|   stm32f0_448_lqfp100 IBIS Model
[IBIS ver]   4.2
[File name]  stm32f0_448_lqfp100.ibs
[File Rev]   1.0
[Date]   15-5-2013
[Source] Data Created at STMicroelectronics
[Notes]   File originated from ELDO simulations.
[Disclaimer]  This information is for modeling purpose only and is
   not guaranted. The information is subject to change without
   notice.
[Copyright] Copyright 2015 STMicroelectronics Inc.
[Component] stm32f0_448_lqfp100
[Manufacturer] STMicroelectronics
[Package]
| variable   typ   min   max
R_pkg   0.0   NA   NA
L_pkg   0.0H   NA   NA
C_pkg   0.0F   NA   NA
[Pin] signal_name  model_name   R_pin   L_pin   C_pin
1   PE2   io8p_sudq_ft   0.132430474   7.03E-09   1.35E-13
2   PE3   io8p_sudq_ft   0.133347678   6.77E-09   1.95E-14
3   PE4   io8p_sudq_ft   0.12897311   6.49E-09   1.04E-14
4   PE5   io8p_sudq_ft   0.125344562   6.21E-09   5.24E-15
5   PE6   io8p_sudq_ft   0.120515446   5.99E-09   7.82E-15
6   VBAT   POWER   0.12047071   5.95E-09   6.53E-15
7   PC13   io8p_sudq_tc   0.117880646   5.78E-09   6.23E-15
8   PC14   io8p_sudq_tc   0.117278614   5.65E-09   3.11E-15
9   PC15   io8p_sudq_tc   0.11554812   5.55E-09   1.39E-15
10   PF9   io8p_sudq_ft   0.114995632   5.43E-09   2.92E-15
11   PF10   io8p_sudq_ft   0.112975638   5.30E-09   3.56E-15
12   PF0   io8p_sudq_ft   0.111323436   5.23E-09   4.78E-15
13   PF1   io8p_sudq_ft   0.109216856   5.14E-09   8.66E-15
14   NRST   ioreset_tc_v33   0.11066442   5.18E-09   9.03E-15
15   PC0   io8p_sudq_ft   0.110607546   5.19E-09   7.98E-15
16   PC1   io8p_sudq_ft   0.111326184   5.25E-09   1.03E-14
17   PC2   io8p_sudq_ft   0.11442005   5.35E-09   7.00E-15
18   PC3   io8p_sudq_ft   0.114363236   5.45E-09   8.65E-15
19   PF2   io8p_sudq_ft   0.117563732   5.62E-09   7.83E-15
20   VSSA   GND   0.119904688   5.80E-09   2.29E-16
21   VDDA   POWER   0.122311852   5.96E-09   1.05E-15
22   PF3   io8p_sudq_ft   0.125384354   6.19E-09   8.12E-16
23   PA0   io8p_sudq_ft   0.129702038   6.49E-09   3.82E-15
24   PA1   io8p_sudq_ft   0.13229018   6.71E-09   6.80E-15
25   PA2   io8p_sudq_ft   0.132955142   7.01E-09   1.67E-14
26   PA3   io8p_sudq_ft   0.13394318   7.05E-09   1.75E-14
27   VSS   GND   0.13495773   6.80E-09   1.27E-14
28   VDD   POWER   0.130511464   6.53E-09   9.83E-15
29   PA4   io8p_sudq_ft   0.1253867   6.24E-09   6.07E-15
30   PA5   io8p_sudq_ft   0.124988978   6.11E-09   5.77E-16
31   PA6   io8p_sudq_ft   0.121784338   5.89E-09   1.52E-15
32   PA7   io8p_sudq_ft   0.119149388   5.72E-09   5.44E-15
33   PC4   io8p_sudq_ft   0.116374808   5.56E-09   4.10E-15
34   PC5   io8p_sudq_ft   0.113278606   5.41E-09   3.69E-15
35   PB0   io8p_sudq_ft   0.112726654   5.36E-09   3.90E-15
36   PB1   io8p_sudq_ft   0.112271006   5.27E-09   1.66E-15
37   PB2   io8p_sudq_ft   0.111816114   5.24E-09   7.92E-15
38   PE7   io8p_sudq_ft   0.110998514   5.18E-09   9.90E-15
39   PE8   io8p_sudq_ft   0.114588522   5.30E-09   7.91E-15
40   PE9   io8p_sudq_ft   0.114461118   5.33E-09   7.94E-15
41   PE10   io8p_sudq_ft   0.11535023   5.42E-09   4.18E-15
42   PE11   io8p_sudq_ft   0.116979452   5.53E-09   6.06E-15
43   PE12   io8p_sudq_ft   0.120184998   5.70E-09   5.12E-15
44   PE13   io8p_sudq_ft   0.12258702   5.87E-09   4.74E-15
45   PE14   io8p_sudq_ft   0.126303358   6.07E-09   1.16E-14
46   PE15   io8p_sudq_ft   0.129714658   6.28E-09   9.91E-15
47   PB10   io8p_sudq_i2cin_lv_ft   0.133373154   6.51E-09   5.08E-15
48   PB11   io8p_sudq_i2cin_lv_ft   0.137888146   6.86E-09   5.47E-15
49   VSS   GND   0.131554082   6.80E-09   4.18E-15
50   VDD   POWER   0.132347744   7.04E-09   1.19E-14
51   PB12   io8p_sudq_ft   0.131767814   7.01E-09   1.62E-14
52   PB13   io8p_sudq_ft   0.131784366   6.75E-09   2.15E-15
53   PB14   io8p_sudq_ft   0.129150704   6.48E-09   9.18E-15
54   PB15   io8p_sudq_ft   0.12519135   6.20E-09   5.66E-15
55   PD8   io8p_sudq_ft   0.121530258   5.99E-09   3.69E-15
56   PD9   io8p_sudq_ft   0.11887369   5.81E-09   7.43E-15
57   PD10   io8p_sudq_ft   0.11586992   5.64E-09   1.06E-14
58   PD11   io8p_sudq_ft   0.113225758   5.47E-09   5.76E-15
59   PD12   io8p_sudq_ft   0.111781608   5.35E-09   6.53E-15
60   PD13   io8p_sudq_ft   0.110712606   5.28E-09   1.14E-14
61   PD14   io8p_sudq_ft   0.110051596   5.20E-09   1.32E-14
62   PD15   io8p_sudq_ft   0.10995365   5.18E-09   1.46E-14
63   PC6   io8p_sudq_ft   0.1097803   5.15E-09   7.25E-15
64   PC7   io8p_sudq_ft   0.112445854   5.26E-09   3.59E-16
65   PC8   io8p_sudq_ft   0.113595842   5.33E-09   6.58E-16
66   PC9   io8p_sudq_ft   0.115707136   5.47E-09   5.09E-16
67   PA8   io8p_sudq_ft   0.116952062   5.60E-09   5.83E-16
68   PA9   io8p_sudq_ft   0.11904328   5.76E-09   5.46E-16
69   PA10   io8p_sudq_ft   0.120673854   5.88E-09   1.39E-14
70   PA11   io8p_sudq_ft   0.124658692   6.11E-09   2.50E-14
71   PA12   io8p_sudq_ft   0.124406978   6.16E-09   3.99E-14
72   PA13   io8p_sudq_ft   0.130155984   6.40E-09   3.02E-13
73   PF6   io8p_sudq_i2cin_lv_ft   0.135109698   6.82E-09   1.55E-13
74   VSS   GND   0.139401952   7.08E-09   1.55E-13
75   VDDIO2  POWER   0.133554014   7.06E-09   3.90E-14
76   PA14   io8p_sudq_ft   0.135294596   7.10E-09   1.63E-14
77   PA15   io8p_sudq_ft   0.132513704   6.84E-09   9.76E-15
78   PC10   io8p_sudq_ft   0.133481516   6.64E-09   9.30E-15
79   PC11   io8p_sudq_ft   0.12836612   6.34E-09   5.42E-15
80   PC12   io8p_sudq_ft   0.124282386   6.09E-09   1.18E-15
81   PD0   io8p_sudq_ft   0.121841172   5.92E-09   5.46E-15
82   PD1   io8p_sudq_ft   0.118487054   5.73E-09   7.00E-15
83   PD2   io8p_sudq_ft   0.117180194   5.57E-09   6.06E-15
84   PD3   io8p_sudq_ft   0.11350052   5.42E-09   5.45E-15
85   PD4   io8p_sudq_ft   0.113789098   5.34E-09   5.29E-16
86   PD5   io8p_sudq_ft   0.110805858   5.26E-09   2.99E-15
87   PD6   io8p_sudq_ft   0.110442376   5.25E-09   2.06E-15
88   PD7   io8p_sudq_ft   0.111525472   5.18E-09   5.68E-15
89   PB3   io8p_sudq_ft   0.11114441   5.22E-09   9.91E-15
90   PB4   io8p_sudq_ft   0.113222316   5.31E-09   9.05E-15
91   PB5   io8p_sudq_ft   0.113322882   5.40E-09   1.29E-14
92   PB6   io8p_sudq_i2cin_lv_ft   0.1158486   5.52E-09   1.26E-14
93   PB7   io8p_sudq_i2cin_lv_ft   0.117577758   5.67E-09   6.14E-15
94   BOOT0   vpp_test_hv   0.1189821   5.80E-09   9.37E-15
95   PB8   io8p_sudq_i2cin_lv_ft   0.121885942   5.96E-09   7.76E-15
96   PB9   io8p_sudq_i2cin_lv_ft   0.126275558   6.16E-09   8.56E-15
97   PE0   io8p_sudq_ft   0.128749356   6.37E-09   8.16E-15
98   PE1   io8p_sudq_ft   0.13328845   6.70E-09   1.03E-15
99   VSS   GND   0.13223018   6.84E-09   4.41E-15
100   VDD   POWER   0.132277204   7.05E-09   1.71E-14
[Model Selector] io8p_sudq_ft
io8p01_sudq_ft_pd_lv  "SPEED01 2P0V, PD=40kOhm"
io8p01_sudq_ft_pu_lv  "SPEED01 2P0V, PU=40kOhm"
io8p01_sudq_ft_lv  "SPEED01 2P0V"
io8p10_sudq_ft_pd_lv  "SPEED10 2P0V, PD=40kOhm"
io8p10_sudq_ft_pu_lv  "SPEED10 2P0V, PU=40kOhm"
io8p10_sudq_ft_lv  "SPEED10 2P0V"
io8p11_sudq_ft_pd_lv  "SPEED11 2P0V, PD=40kOhm"
io8p11_sudq_ft_pu_lv  "SPEED11 2P0V, PU=40kOhm"
io8p11_sudq_ft_lv  "SPEED11 2P0V"
io8p01_sudq_ft_pd  "SPEED01, PD=40kOhm"
io8p01_sudq_ft_pu  "SPEED01, PU=40kOhm"
io8p01_sudq_ft  "SPEED01"
io8p10_sudq_ft_pd  "SPEED10, PD=40kOhm"
io8p10_sudq_ft_pu  "SPEED10, PU=40kOhm"
io8p10_sudq_ft  "SPEED10"
io8p11_sudq_ft_pd  "SPEED11, PD=40kOhm"
io8p11_sudq_ft_pu  "SPEED11, PU=40kOhm"
io8p11_sudq_ft  "SPEED11"
[Model Selector] io8p_sudq_i2cin_lv_ft
io8p01_sudq_i2cin_lv_ft_pd_lv  "SPEED01 2P0V, PD=40kOhm"
io8p01_sudq_i2cin_lv_ft_pu_lv  "SPEED01 2P0V, PU=40kOhm"
io8p01_sudq_i2cin_lv_ft_lv  "SPEED01 2P0V"
io8p10_sudq_i2cin_lv_ft_pd_lv  "SPEED10 2P0V, PD=40kOhm"
io8p10_sudq_i2cin_lv_ft_pu_lv  "SPEED10 2P0V, PU=40kOhm"
io8p10_sudq_i2cin_lv_ft_lv  "SPEED10 2P0V"
io8p11_sudq_i2cin_lv_ft_pd_lv  "SPEED11 2P0V, PD=40kOhm"
io8p11_sudq_i2cin_lv_ft_pu_lv  "SPEED11 2P0V, PU=40kOhm"
io8p11_sudq_i2cin_lv_ft_lv  "SPEED11 2P0V"
io8p01_sudq_i2cin_lv_ft_pd  "SPEED01, PD=40kOhm"
io8p01_sudq_i2cin_lv_ft_pu  "SPEED01, PU=40kOhm"
io8p01_sudq_i2cin_lv_ft  "SPEED01"
io8p10_sudq_i2cin_lv_ft_pd  "SPEED10, PD=40kOhm"
io8p10_sudq_i2cin_lv_ft_pu  "SPEED10, PU=40kOhm"
io8p10_sudq_i2cin_lv_ft  "SPEED10"
io8p11_sudq_i2cin_lv_ft_pd  "SPEED11, PD=40kOhm"
io8p11_sudq_i2cin_lv_ft_pu  "SPEED11, PU=40kOhm"
io8p11_sudq_i2cin_lv_ft  "SPEED11"
[Model Selector] io8p_sudq_tc
io8p01_sudq_tc_pd_lv  "SPEED01 2P0V, PD=40kOhm"
io8p01_sudq_tc_pu_lv  "SPEED01 2P0V, PU=40kOhm"
io8p01_sudq_tc_lv  "SPEED01 2P0V"
io8p10_sudq_tc_pd_lv  "SPEED10 2P0V, PD=40kOhm"
io8p10_sudq_tc_pu_lv  "SPEED10 2P0V, PU=40kOhm"
io8p10_sudq_tc_lv  "SPEED10 2P0V"
io8p11_sudq_tc_pd_lv  "SPEED11 2P0V, PD=40kOhm"
io8p11_sudq_tc_pu_lv  "SPEED11 2P0V, PU=40kOhm"
io8p11_sudq_tc_lv  "SPEED11 2P0V"
io8p01_sudq_tc_pd  "SPEED01, PD=40kOhm"
io8p01_sudq_tc_pu  "SPEED01, PU=40kOhm"
io8p01_sudq_tc  "SPEED01"
io8p10_sudq_tc_pd  "SPEED10, PD=40kOhm"
io8p10_sudq_tc_pu  "SPEED10, PU=40kOhm"
io8p10_sudq_tc  "SPEED10"
io8p11_sudq_tc_pd  "SPEED11, PD=40kOhm"
io8p11_sudq_tc_pu  "SPEED11, PU=40kOhm"
io8p11_sudq_tc  "SPEED11"
[Model Selector] ioreset_tc_v33
ioreset_tc_v33_pu_lv  "IORESET 2V + PU=40kOhm"
ioreset_tc_v33_nopu_lv  "IORESET 2V"
ioreset_tc_v33_pu  "IORESET + PU=40kOhm"
ioreset_tc_v33_nopu  "IORESET"
[Model Selector] vpp_test_hv
vpp_test_hv_3p3  "Input Buffer"
vpp_test_hv_2p4  "Input Buffer 2P0V"
| Models and submodels in the file (60): io8p01_sudq_ft_pd_lv (I/O), io8p01_sudq_ft_pu_lv (I/O), io8p01_sudq_ft_lv (I/O), io8p10_sudq_ft_pd_lv (I/O), io8p10_sudq_ft_pu_lv (I/O), io8p10_sudq_ft_lv (I/O), io8p11_sudq_ft_pd_lv (I/O), io8p11_sudq_ft_pu_lv (I/O), io8p11_sudq_ft_lv (I/O), io8p01_sudq_ft_pd (I/O), io8p01_sudq_ft_pu (I/O), io8p01_sudq_ft (I/O), io8p10_sudq_ft_pd (I/O), io8p10_sudq_ft_pu (I/O), io8p10_sudq_ft (I/O), io8p11_sudq_ft_pd (I/O), io8p11_sudq_ft_pu (I/O), io8p11_sudq_ft (I/O), io8p01_sudq_i2cin_lv_ft_pd_lv (I/O), io8p01_sudq_i2cin_lv_ft_pu_lv (I/O), io8p01_sudq_i2cin_lv_ft_lv (I/O), io8p10_sudq_i2cin_lv_ft_pd_lv (I/O), io8p10_sudq_i2cin_lv_ft_pu_lv (I/O), io8p10_sudq_i2cin_lv_ft_lv (I/O), io8p11_sudq_i2cin_lv_ft_pd_lv (I/O), io8p11_sudq_i2cin_lv_ft_pu_lv (I/O), io8p11_sudq_i2cin_lv_ft_lv (I/O), io8p01_sudq_i2cin_lv_ft_pd (I/O), io8p01_sudq_i2cin_lv_ft_pu (I/O), io8p01_sudq_i2cin_lv_ft (I/O), io8p10_sudq_i2cin_lv_ft_pd (I/O), io8p10_sudq_i2cin_lv_ft_pu (I/O), io8p10_sudq_i2cin_lv_ft (I/O), io8p11_sudq_i2cin_lv_ft_pd (I/O), io8p11_sudq_i2cin_lv_ft_pu (I/O), io8p11_sudq_i2cin_lv_ft (I/O), io8p01_sudq_tc_pd_lv (I/O), io8p01_sudq_tc_pu_lv (I/O), io8p01_sudq_tc_lv (I/O), io8p10_sudq_tc_pd_lv (I/O), io8p10_sudq_tc_pu_lv (I/O), io8p10_sudq_tc_lv (I/O), io8p11_sudq_tc_pd_lv (I/O), io8p11_sudq_tc_pu_lv (I/O), io8p11_sudq_tc_lv (I/O), io8p01_sudq_tc_pd (I/O), io8p01_sudq_tc_pu (I/O), io8p01_sudq_tc (I/O), io8p10_sudq_tc_pd (I/O), io8p10_sudq_tc_pu (I/O), io8p10_sudq_tc (I/O), io8p11_sudq_tc_pd (I/O), io8p11_sudq_tc_pu (I/O), io8p11_sudq_tc (I/O), ioreset_tc_v33_pu_lv (I/O_open_drain), ioreset_tc_v33_nopu_lv (I/O_open_drain), ioreset_tc_v33_pu (I/O_open_drain), ioreset_tc_v33_nopu (I/O_open_drain), vpp_test_hv_2p4 (Input), vpp_test_hv_3p3 (Input)
